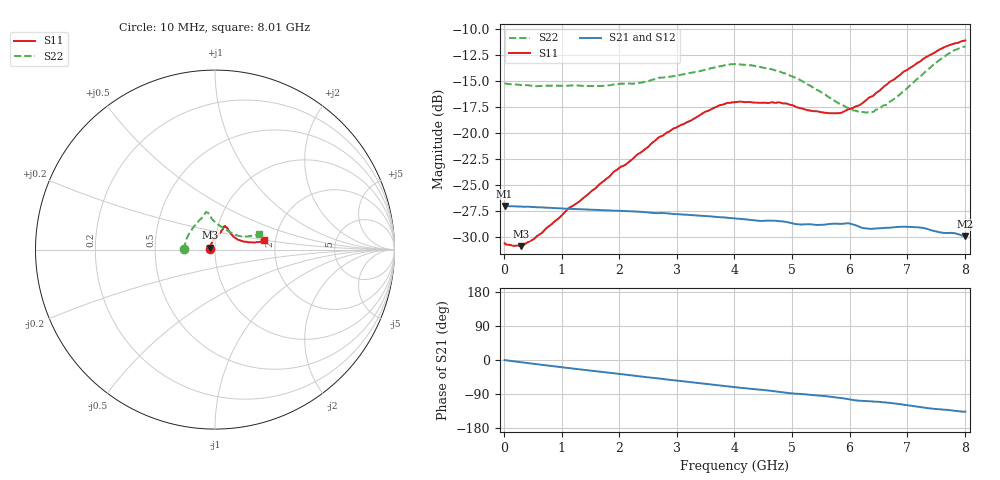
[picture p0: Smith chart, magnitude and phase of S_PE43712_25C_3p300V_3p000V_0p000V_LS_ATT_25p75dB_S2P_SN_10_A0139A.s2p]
! DEVICE ID: PE43712
! File Path: z:\PE43713\PE43713_CHAR_NOM_04292014\AMB\3p300\LS_ATT_25p75dB\PE43713_AMB_3p300V_3p000V_0p000V_LS_ATT_25p75dB_S2P_SN_10_A0139A.s2p
! Serial: 10
! Lot: A0139A
! Temp: 25C
! VDD: 3.300
! VSS: 0.000
! Control_Hi: 3.000
! Control_Lo: 0.000
! Attenuation Step: 25.75dB
! Port 1: RF1
! Port 2: RF2
! ThroughPath:1-2
! IDD: 0.0001452815
! ISS: -9.22e-008
#  Hz  S  RI  R  50
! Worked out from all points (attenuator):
!   801 points, 10 MHz to 8.01 GHz, reference 50 ohm
!   highest |S21| = -27.01 dB at 10 MHz (marker M1); lowest = -29.9 dB at 8.01 GHz (marker M2)
!   lowest |S11| = -30.9 dB at 290 MHz (marker M3), VSWR 1.06, Z = 47.4 + j1.03 ohm
!   |S11| at or under -10 dB: start of sweep to end of sweep
!   |S22| runs from -18.0 to -11.6 dB; largest |S21 - S12| = 0.00018
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1e7  -0.0296 0.000802  0.0446 -0.000205  0.0446 -0.000186  -0.1738 0.00124
2.9e8  -0.0264 0.0109  0.0441 -0.00449  0.0442 -0.00448  -0.1697 0.0197
6.4e8  -0.0234 0.0231  0.0429 -0.00948  0.0429 -0.00949  -0.1635 0.0415
1.12e9  -0.0179 0.0397  0.0404 -0.0157  0.0404 -0.0157  -0.1541 0.0711
1.35e9  -0.0133 0.0462  0.0389 -0.0184  0.0389 -0.0184  -0.1473 0.0833
1.91e9  0.000812 0.0654  0.0347 -0.0244  0.0347 -0.0244  -0.1259 0.1171
2.27e9  0.0128 0.0761  0.0314 -0.0279  0.0314 -0.0279  -0.1096 0.1346
2.68e9  0.0267 0.0915  0.0273 -0.0309  0.0273 -0.0309  -0.0888 0.1621
3.5e9  0.0458 0.1186  0.0182 -0.0356  0.0181 -0.0356  -0.0594 0.1935
3.74e9  0.0496 0.1271  0.0154 -0.0363  0.0154 -0.0363  -0.0552 0.2028
4.01e9  0.0534 0.131  0.0123 -0.0369  0.0123 -0.0369  -0.0523 0.2089
4.75e9  0.0636 0.1256  0.0042 -0.0376  0.00422 -0.0376  -0.0326 0.1974
5.35e9  0.0803 0.0998  -0.00159 -0.0363  -0.00161 -0.0363  -0.0141 0.1667
5.81e9  0.1006 0.0741  -0.00628 -0.0361  -0.00622 -0.0361  0.0195 0.1379
5.99e9  0.113 0.0657  -0.00877 -0.0358  -0.00869 -0.0358  0.0366 0.1272
6.17e9  0.1241 0.0568  -0.0106 -0.0337  -0.0106 -0.0338  0.0554 0.1134
6.4e9  0.1424 0.0503  -0.0114 -0.0327  -0.0113 -0.0327  0.0815 0.097
6.68e9  0.1698 0.0436  -0.0137 -0.0323  -0.0136 -0.0323  0.1146 0.0816
7.17e9  0.2139 0.0399  -0.0192 -0.0297  -0.0191 -0.0296  0.1668 0.0736
7.56e9  0.2492 0.0436  -0.0215 -0.0255  -0.0215 -0.0255  0.2114 0.0784
7.81e9  0.2659 0.0481  -0.0228 -0.0239  -0.0229 -0.0239  0.2358 0.084
8.01e9  0.2751 0.0521  -0.023 -0.022  -0.023 -0.0221  0.2476 0.0849
